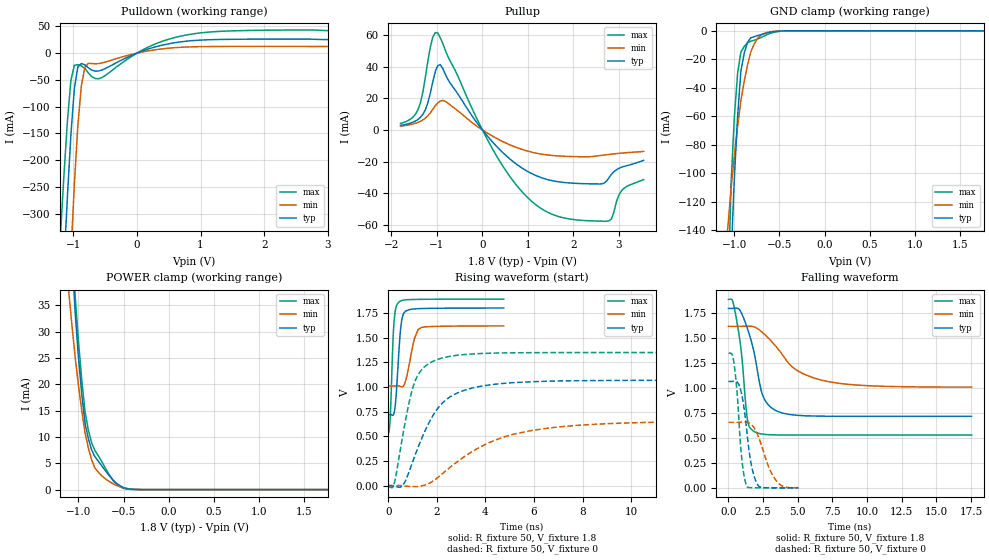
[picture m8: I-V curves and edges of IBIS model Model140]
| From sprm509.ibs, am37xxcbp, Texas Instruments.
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| Model based on original model for DSIPHY_WIO_ADDON_GPIOWRAPPER
|   Sub model PB_HS10L10_PUPD0_1P8
[model]   Model140
|[Input Load]   PI
|[Output Drive] SC10LB10
|Voltage   1.8V
|Mode   I/O
Model_type   I/O
Polarity   Non-Inverting
Enable   Active-Low
Vinl =  0.63
Vinh =  1.17
Cref =  15pF
Rref =  100.0000M
Vref =  0V
Vmeas =  0.9
C_comp   1.429432p   1.270657p   1.602015p
[Model Spec]
Vinl   0.63   0.567   0.6615
Vinh   1.17   1.053   1.2285
[Temperature Range]   25   125   -40
[Voltage Range]   1.8   1.62   1.89
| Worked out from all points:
|   slope of the pulldown table from 0 to 0.27 V, typ, clamps not added: 24.3 ohm
|   slope of the pullup table from 0 to 0.27 V, typ, clamps not added: 29.7 ohm
|   GND clamp passes 1 mA (typ) near -0.60 V on its own axis
|   POWER clamp passes 1 mA (typ) near -0.56 V on its own axis
|   rising waveform, R_fixture 50, V_fixture 1.8: 20-80 % time 177ps typ, 306ps min, 125ps max; typ from 0.717 V to 1.8 V
|   rising waveform, R_fixture 50, V_fixture 0: 20-80 % time 1.34ns typ, 2.95ns min, 708ps max; typ from 0 V to 1.07 V
|   falling waveform, R_fixture 50, V_fixture 1.8: 20-80 % time 1.06ns typ, 2.68ns min, 601ps max; typ from 1.8 V to 0.718 V
|   falling waveform, R_fixture 50, V_fixture 0: 20-80 % time 611ps typ, 1.04ns min, 434ps max; typ from 1.07 V to 0 V
[POWER_clamp]
-1.8V     362.5mA    191.4mA    412.8mA
-1.109V   56.69mA    37.71mA    60.38mA
-1.073V   44.6mA     31.22mA    47.8mA
-1.036V   33.44mA    25.04mA    36.59mA
-1V       24.98mA    19.72mA    28.06mA
-963.6mV  18.03mA    14.96mA    20.78mA
-927.3mV  12.59mA    10.77mA    14.74mA
-890.9mV  9.653mA    7.899mA    11.31mA
-818.2mV  6.214mA    4.114mA    7.414mA
-636.4mV  2.183mA    1.307mA    2.238mA
-418.2mV  83.85uA    105.2uA    35.14uA
1.764V    -1.228nA   -79.12nA   -1.453nA
[Pulldown]
-1.8V     -1.718A    -2.61A     -1.406A
-1.2V     -527.4mA   -844.5mA   -339.9mA
-1.145V   -396mA     -683.1mA   -229.1mA
-1.091V   -269mA     -526.7mA   -127.5mA
-1.036V   -153.6mA   -378.9mA   -51.17mA
-981.8mV  -66.34mA   -245.6mA   -22.67mA
-927.3mV  -26mA      -136.2mA   -21.54mA
-872.7mV  -19.34mA   -61.98mA   -23.69mA
-763.6mV  -27.2mA    -19.05mA   -36.72mA
-545.5mV  -31.39mA   -18.17mA   -45.46mA
872.7mV   23.46mA    11.88mA    35.92mA
3.545V    25.34mA    12.51mA    41.58mA
[Pullup]
-1.8V     2.903mA    2.423mA    4.112mA
-1.418V   6.595mA    4.711mA    12.64mA
-1.255V   12.69mA    7.42mA     33.23mA
-1.091V   30.4mA     13mA       58.69mA
-981.8mV  40.63mA    17.02mA    61.3mA
-818.2mV  35.38mA    18.12mA    50.59mA
272.7mV   -9.18mA    -4.728mA   -14.55mA
1.255V    -29.75mA   -15.09mA   -48.97mA
2.564V    -34.17mA   -16.31mA   -57.57mA
2.782V    -30.25mA   -15.5mA    -57.48mA
3.055V    -23.63mA   -14.68mA   -38.61mA
3.545V    -19.25mA   -13.56mA   -31.41mA
[GND_clamp]
-1.8V     -2.82A     -1.192A    -3.165A
-1.073V   -235.7mA   -138.4mA   -192.1mA
-1.036V   -159.5mA   -110.8mA   -107.5mA
-1V       -103.8mA   -87.85mA   -60.67mA
-963.6mV  -60mA      -67.28mA   -29.8mA
-927.3mV  -28.21mA   -49.08mA   -14.9mA
-890.9mV  -15.9mA    -35.48mA   -10.99mA
-854.5mV  -8.138mA   -24.07mA   -8.449mA
-818.2mV  -4.924mA   -14.85mA   -7.266mA
-709.1mV  -2.784mA   -3.064mA   -4.883mA
-563.6mV  -570.2uA   -404.5uA   -1.092mA
1.764V    -11.02pA   583.5nA    3.035nA
[Ramp]
dV/dt_f  0.6514386/1.056371n   0.3679504/2.702819n   0.8183712/0.6029826n
dV/dt_r  0.6511092/1.344502n   0.4007838/2.979439n   0.8230479/0.709531n
R_load = 50
[Rising Waveform]
R_fixture = 50
V_fixture = 1.8
V_fixture_min = 1.62
V_fixture_max = 1.89
0s        717.3mV    1.009V     528.5mV
81ps      718.9mV    1.009V     711.8mV
180ps     711.9mV    1.009V     1.408V
234ps     736mV      1.009V     1.66V
396ps     1.208V     1.011V     1.849V
522ps     1.629V     1.003V     1.873V
729ps     1.77V      1.079V     1.883V
1.071ns   1.79V      1.488V     1.887V
1.377ns   1.795V     1.603V     1.888V
4.752ns   1.8V       1.618V     1.89V
[Rising Waveform]
R_fixture = 50
V_fixture = 0
V_fixture_min = 0
V_fixture_max = 0
0s        -197uV     102.1uV    -10.3mV
234ps     -8.544mV   -227.2uV   13.41mV
612ps     8.669mV    -2.778mV   534.2mV
891ps     167.2mV    -8.016mV   881.7mV
1.125ns   324.3mV    -10.54mV   1.074V
1.701ns   651mV      25.47mV    1.242V
2.232ns   838.7mV    121.9mV    1.294V
4.203ns   1.022V     440.6mV    1.342V
6.48ns    1.057V     579.7mV    1.348V
20.3ns    1.067V     655.8mV    1.349V
[Falling Waveform]
R_fixture = 50
V_fixture = 1.8
V_fixture_min = 1.62
V_fixture_max = 1.89
0s        1.8V       1.62V      1.89V
315ps     1.801V     1.62V      1.869V
738ps     1.796V     1.62V      1.561V
1.377ns   1.595V     1.622V     679.4mV
1.845ns   1.361V     1.615V     565.9mV
2.592ns   889.9mV    1.542V     537mV
3.852ns   752.4mV    1.343V     530.4mV
5.112ns   726.6mV    1.165V     529.8mV
7.578ns   718.3mV    1.057V     529.8mV
17.54ns   717.6mV    1.011V     529.8mV
[Falling Waveform]
R_fixture = 50
V_fixture = 0
V_fixture_min = 0
V_fixture_max = 0
0s        1.068V     657.4mV    1.349V
243ps     1.068V     657.6mV    1.345V
405ps     1.071V     657.4mV    1.245V
612ps     1.063V     657.4mV    975.5mV
972ps     925.6mV    659.9mV    277.4mV
1.314ns   583.1mV    659.3mV    19.27mV
1.665ns   220.5mV    633.4mV    1.754mV
2.187ns   16.81mV    505.5mV    212.6uV
3.474ns   354.2uV    67.93mV    5.749uV
5.04ns    57.44uV    1.639mV    669.3nV
